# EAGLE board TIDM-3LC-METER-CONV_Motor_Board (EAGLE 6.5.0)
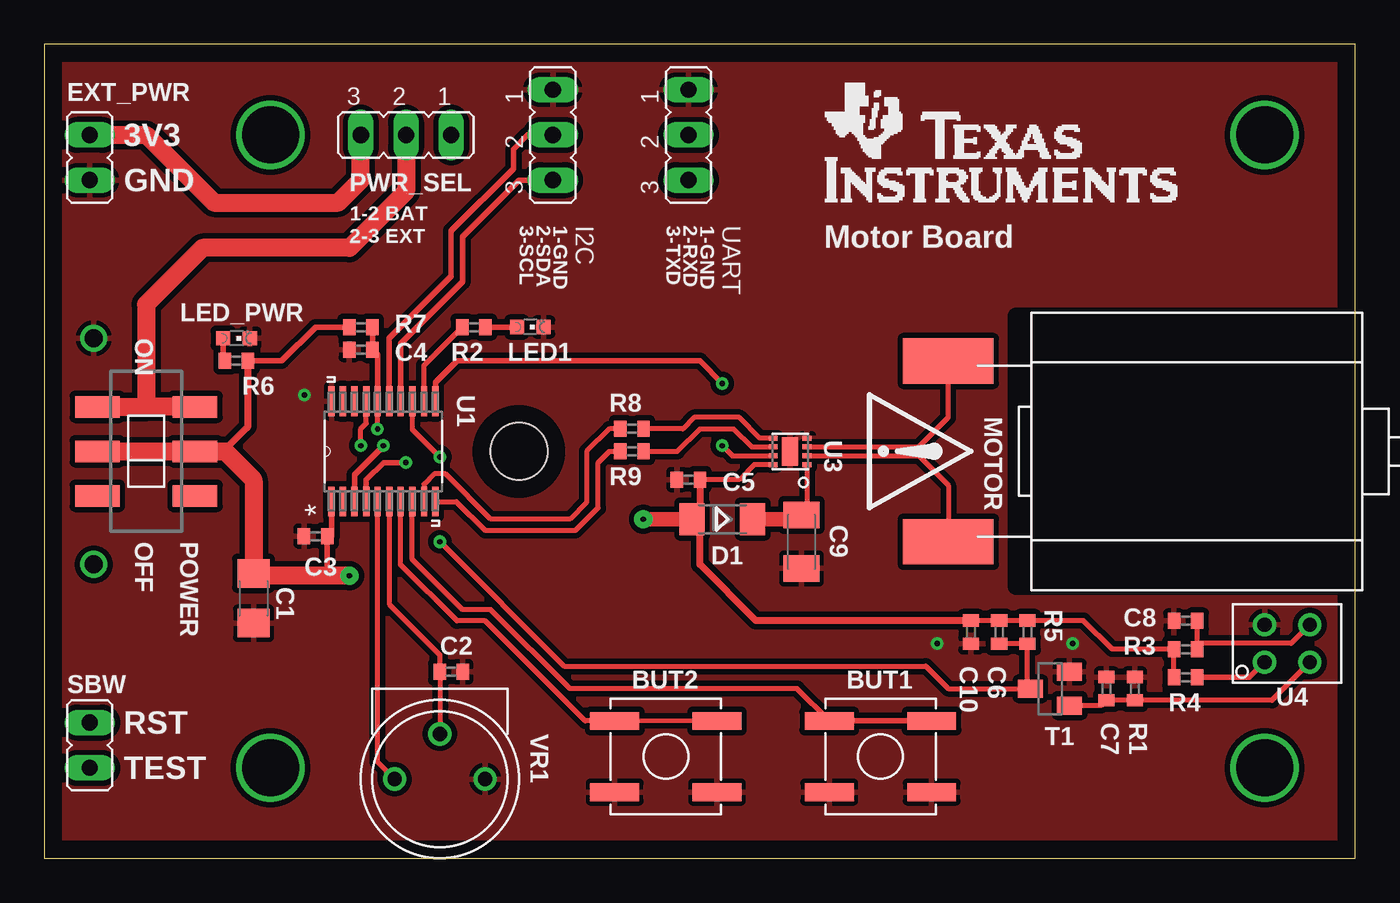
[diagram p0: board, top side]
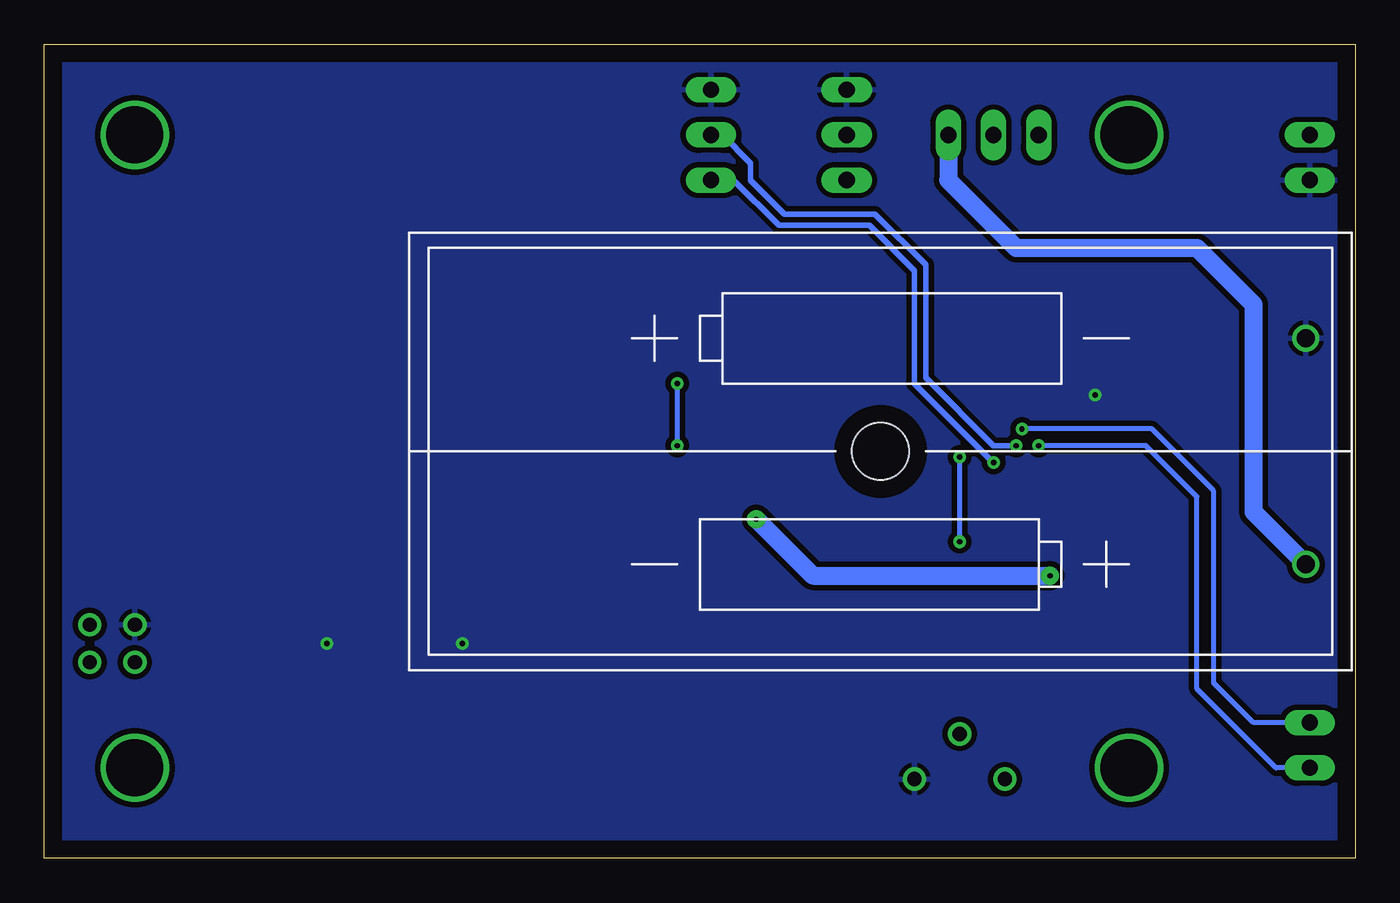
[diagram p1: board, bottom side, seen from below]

Size 73.66 x 45.72 mm. Coordinates in mm from the lower left corner, seen from the top.
Outline: 73.66,45.72 0,45.72 0,0 73.66,0 73.66,45.72
Copper layers (1*16): Top 0.035mm / dielectric 1.5mm / Bottom 0.035mm
Design rules "default *": minimum track width 6mil, minimum drill 0.3mm, track to track 6mil, track to pad 6mil, pad to pad 6mil, via to via 6mil, smd to smd 6mil, copper to edge 1mm, drill to drill 8mil, minimum pad ring 10mil, minimum via ring 8mil, stop-mask expansion 4mil, vias tented up to drill 100mil, thermal gap 10mil
tRestrict: area 54.6,15.2 to 73.7,30.5

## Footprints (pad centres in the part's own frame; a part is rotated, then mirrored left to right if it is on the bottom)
2X3A(1_HOLE) = drill 1: + 23.901,-6.35; - 23.901,6.35 | hole 3.2: 0,0
BUT = smd 2.75 x 1: P$1 2.875,-2; P$2 -2.875,-2; P$3 2.875,2; P$4 -2.875,2
C1206 = smd 1.6 x 1.8: 1 -1.4,0; 2 1.4,0
C0402 = smd 0.7 x 0.9: 1 -0.65,0; 2 0.65,0
C1206K = smd 1.5 x 2: 1 -1.5,0; 2 1.5,0
SOD80 = smd 1.4 x 1.8: 1 -1.7,0; 2 1.7,0
JP1 = drill 0.914 long: 1 0,-1.27; 2 0,1.27
JP2 = drill 0.914 long: 1 -2.54,0; 2 0,0; 3 2.54,0
CHIPLED_0603 = smd 0.8 x 0.8: A 0,-0.75; C 0,0.75
MOTOR = smd 5.08 x 2.54: + 13.97,5.08; - 13.97,-5.08
2P2T = smd 1.2 x 2.5: 1 -2.5,2.75; 2 0,2.75; 3 2.5,2.75; 4 -2.5,-2.75; 5 0,-2.75; 6 2.5,-2.75
R0402 = smd 0.7 x 0.9: 1 -0.65,0; 2 0.65,0
SOT23-BEC = smd 1 x 1.4: B -0.95,-1.1; C 0,1.1; E 0.95,-1.1
PW20 = smd 1.676 x 0.356: 1 -2.819,2.921; 2 -2.819,2.286; 3 -2.819,1.626; 4 -2.819,0.965; 5 -2.819,0.33; 6 -2.819,-0.33; 7 -2.819,-0.965; 8 -2.819,-1.626; 9 -2.819,-2.286; 10 -2.819,-2.921; 11 2.819,-2.921; 12 2.819,-2.286; 13 2.819,-1.626; 14 2.819,-0.965; 15 2.819,-0.33; 16 2.819,0.33; 17 2.819,0.965; 18 2.819,1.626; 19 2.819,2.286; 20 2.819,2.921
DSG-S-PWSON-N8 = smd 0.28 x 0.5: 1 -0.75,-0.95; 2 -0.25,-0.95; 3 0.25,-0.95; 4 0.75,-0.95; 5 0.75,0.95; 6 0.25,0.95; 7 -0.25,0.95; 8 -0.75,0.95 | smd 1.6 x 0.9: P$9 0,0
CUSTOM_4L = drill 0.8: P1 -1.054,1.27; P2 -1.054,-1.27; P3 1.054,-1.27; P4 1.054,1.27
3352P = drill 0.8: 1 -2.54,0; 2 0,-2.54; 3 2.54,0

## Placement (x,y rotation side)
BAT1  2XAAA-1  [2X3A(1_HOLE)]  26.67,22.86 0 bottom
BUT1  B3SL-1002P  [BUT]  46.99,5.71 0 top
BUT2  B3SL-1002P  [BUT]  34.92,5.71 0 top
C1  22uF  [C1206]  11.75,14.61 270 top
C2  100nF  [C0402]  22.86,10.48 0 top
C3  100nF  [C0402]  15.24,18.1 180 top
C4  2n2  [C0402]  17.78,28.57 180 top
C5  100nF  [C0402]  36.2,21.27 180 top
C6  470nF  [C0402]  53.66,12.7 270 top
C7  100nF  [C0402]  59.69,9.53 90 top
C8  100nF  [C0402]  64.14,13.34 180 top
C9  22uF  [C1206K]  42.55,17.78 270 top
C10  100nF  [C0402]  52.07,12.7 270 top
D1  FDLL4148  [SOD80]  38.1,19.05 180 top
EXT_PWR  [JP1]  2.54,39.37 180 top
I2C  [JP2]  28.57,40.64 270 top
LED1  [CHIPLED_0603]  27.3,29.84 270 top
LED_PWR  [CHIPLED_0603]  10.79,29.21 270 top
MOTOR  MOTOR  [MOTOR]  64.77,22.86 180 top
POWER  2P2T  [2P2T]  5.71,22.86 90 top
PWR_SEL  [JP2]  20.32,40.64 180 top
R1  10K  [R0402]  61.28,9.53 270 top
R2  470R  [R0402]  24.13,29.84 180 top
R3  1K  [R0402]  64.14,11.75 180 top
R4  100R  [R0402]  64.14,10.16 180 top
R5  2K  [R0402]  55.24,12.7 270 top
R6  470R  [R0402]  10.79,27.94 0 top
R7  47K  [R0402]  17.78,29.84 180 top
R8  100R  [R0402]  33.02,24.13 180 top
R9  100R  [R0402]  33.02,22.86 180 top
SBW  [JP1]  2.54,6.35 0 top
T1  [SOT23-BEC]  56.52,9.53 90 top
U1  MSP430G2333_PW_20  [PW20]  19.05,22.86 90 top
U3  DRV8837DSG  [DSG-S-PWSON-N8]  41.91,22.86 90 top
U4  QRD1113  [CUSTOM_4L]  69.85,12.06 90 top
U$1  TI-LOGO-SMALL  [TI-LOGO-4]  43.81,36.7 0 top
UART  [JP2]  36.2,40.64 270 top
VR1  3352P  [3352P]  22.23,4.45 180 top

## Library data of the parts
BAT1 = battery
BUT1 BUT2 = Button
C1-C10 R1-R9 = rcl
D1 = semicon-smd-ipc
EXT_PWR I2C PWR_SEL SBW UART = jumper
LED1 LED_PWR = led
MOTOR = motor
POWER = switch
T1 = transistor
U1 = MSP430; DATASHEETURL: http://www.ti.com/lit/gpn/MSP430G2333; DESCRIPTION: MSP430G2x33, MSP430G2x03 Mixed Signal Microcontroller; FAMILY_NAME: Value Line; GENERIC_PART_NUMBER: MSP430G2333; INDUSTRY_STD_PKG_TYPE: TSSOP; MANUFACTURER: Texas Instruments; MANUFACTURER_PART_NUMBER: msp430g2333_pw_20; PACKAGE_DESIGNATOR: PW; PIN_COUNT: 20; VENDOR: Texas Instruments
U3 = Motor Driver
U4 = Opto-Sensor
U$1 = texas-logo
VR1 = Trimmer

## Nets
BUT1: BUT1.P$3 BUT1.P$4 U1.8
BUT2: BUT2.P$3 BUT2.P$4 U1.7
GND: BAT1.- BUT1.P$1 BUT1.P$2 BUT2.P$1 BUT2.P$2 C1.2 C2.2 C3.2 C4.2 C5.2 C7.2 C8.2 C9.2 C10.2 EXT_PWR.2 I2C.1 LED1.C LED_PWR.C R1.1 T1.E U1.20 U3.4 U3.P$9 U4.P4 UART.1 VR1.1
LED: R2.2 U1.12
MOTOR_PWM1: R9.1 U3.6
MOTOR_PWM2: R8.1 U3.5
N$1: LED1.A R2.1
N$2: MOTOR.+ U3.2
N$3: C7.1 R1.2 T1.B U4.P2
N$4: MOTOR.- U3.3
N$5: R4.1 U4.P1
N$6: R8.2 U1.9
N$7: C9.1 D1.1 U3.1
N$8: R9.2 U1.10
N$10: C8.1 R3.1 U4.P3
N$13: BAT1.+ PWR_SEL.1
N$14: EXT_PWR.1 PWR_SEL.3
N$15: POWER.3 POWER.6 PWR_SEL.2
N$18: LED_PWR.A R6.1
ROT1: C6.2 R5.2 T1.C U1.13
RST/SBWTDIO: C4.1 R7.1 SBW.2 U1.16
RXD: U1.3 UART.2
SCL: I2C.3 U1.14
SDA: I2C.2 U1.15
SLEEP: U1.11 U3.7
TEST/SBWTCK: SBW.1 U1.17
TXD: U1.4 UART.3
VCC: C1.1 C3.1 C5.1 C6.1 C10.1 D1.2 POWER.2 POWER.5 R3.2 R4.2 R5.1 R6.2 R7.2 U1.1 U3.8
VRIN: C2.1 U1.6 VR1.2
VROUT: U1.5 VR1.3

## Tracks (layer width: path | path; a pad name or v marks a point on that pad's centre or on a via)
BUT1
  Top 0.279: BUT1.P$4 42.3,9.53 29.53,9.53 25.08,13.97 23.5,13.97 20.68,16.79 U1.8
  Top 0.305: BUT1.P$3 BUT1.P$4
BUT2
  Top 0.254: BUT2.P$4 BUT2.P$3 36.83,7.71
  Top 0.279: U1.7 20.02,16.5 23.18,13.34 24.77,13.34 30.39,7.71 BUT2.P$4
GND  (via drill 0.3)
  other vias: 50.16,12.06 57.78,12.06 14.61,26.04
  pour Bottom (isolate 0.305): 73.66,0 0,0 0,45.72 73.66,45.72
  pour Top (isolate 0.305): 73.66,45.72 0,45.72 0,0 73.66,0
LED
  Top 0.279: U1.12 21.34,27.69 R2.2
MOTOR_PWM1
  Top 0.279: R9.1 35.56,22.86 36.83,24.13 38.73,24.13 39.76,23.11 U3.6
MOTOR_PWM2
  Top 0.279: U3.5 40.21,23.61 39.05,24.77 36.51,24.77 35.88,24.13 R8.1
N$1
  Top 0.305: R2.1 LED1.A
N$2
  Top 0.279: U3.2 49.15,22.61 50.8,20.95 MOTOR.+
N$3
  Top 0.279: U4.P2 68.98,8.88 R1.2 C7.1 59.39,8.57 T1.B
N$4
  Top 0.279: U3.3 49.15,23.11 50.8,24.77 MOTOR.-
N$5
  Top 0.305: U4.P1 67.73,10.16 R4.1
N$6
  Top 0.279: R8.2 31.75,24.13 30.48,22.86 30.48,20 29.53,19.05 25.08,19.05 22.54,21.59 21.91,21.59 21.34,21.02 U1.9
N$7
  Top 0.279: U3.1 42.86,19.59 C9.1
  Top 0.813: D1.1 42.31,19.05 C9.1
N$8
  Top 0.279: U1.10 23.14,20.04 24.77,18.41 29.84,18.41 31.11,19.68 31.11,22.23 31.75,22.86 R9.2 32.38,22.84
N$10
  Top 0.279: C8.1 R3.1 64.78,12.06 70.07,12.06 U4.P3
N$13
  Bottom 1.016: PWR_SEL.1 22.86,38.1 19.05,34.29 8.89,34.29 5.71,31.11 5.71,19.46 BAT1.+
N$14
  Top 1.016: EXT_PWR.1 5.71,40.64 9.53,36.83 16.51,36.83 17.78,38.1 PWR_SEL.3
N$15
  Top 1.016: PWR_SEL.2 20.32,37.47 17.14,34.29 8.89,34.29 5.71,31.11 5.71,25.4 | 5.71,25.4 8.43,25.4 POWER.6 | POWER.3 5.67,25.36 5.71,25.4
N$16  (via drill 3.2)
  other vias: 12.7,40.64
N$17  (via drill 3.2)
  other vias: 12.7,5.08
N$18
  Top 0.305: R6.1 10.12,27.97 arc-45 10.04,28.14 LED_PWR.A
N$20  (via drill 3.2)
  other vias: 68.58,5.08
N$21  (via drill 3.2)
  other vias: 68.58,40.64
ROT1  (via drill 0.3)
  Top 0.279: C6.2 R5.2 55.24,9.7 T1.C 50.8,9.53 49.53,10.79 29.21,10.79 v22.23,17.78 | U1.13 20.68,24.09 v22.23,22.54
  Bottom 0.279: v22.23,22.54 v22.23,17.78
RST/SBWTDIO  (via drill 0.3)
  Top 0.279: v18.72,24.12 U1.16
  Top 0.305: U1.16 18.72,28.29 C4.1 R7.1
  Bottom 0.279: SBW.2 5.71,7.62 7.94,9.84 7.94,20.64 11.42,24.12 v18.72,24.12
RXD  (via drill 0.3)
  Top 0.305: v19.05,23.18 17.42,21.55 U1.3
  Bottom 0.305: v19.05,23.18 20.32,23.18 24.13,26.99 24.13,33.34 26.99,36.2 32.07,36.2 33.97,38.1 33.97,39.05 35.56,40.64 UART.2
SCL
  Top 0.305: U1.14 20.02,28.91 23.5,32.38 23.5,34.92 26.67,38.1 I2C.3
SDA
  Top 0.305: U1.15 19.38,29.22 22.86,32.7 22.86,35.24 26.35,38.73 26.35,39.85 27.15,40.64 I2C.2
SLEEP  (via drill 0.3)
  Top 0.279: v38.1,23.18 38.67,22.61 U3.7
  Top 0.305: U1.11 21.97,26.73 23.18,27.94 36.83,27.94 v38.1,26.67
  Bottom 0.279: v38.1,26.67 v38.1,23.18
TEST/SBWTCK  (via drill 0.3)
  Top 0.279: v17.78,23.18 17.78,24.13 18.09,24.43 U1.17
  Bottom 0.279: SBW.1 4.45,5.08 8.89,9.53 8.89,20.32 11.75,23.18 v17.78,23.18
TXD  (via drill 0.3)
  Top 0.305: v20.32,22.23 19.05,22.23 18.09,21.26 U1.4
  Bottom 0.305: UART.3 34.92,38.1 32.38,35.56 27.3,35.56 24.77,33.02 24.77,26.67 v20.32,22.23
VCC  (via drill 0.3 pad 1.02)
  Top 0.279: R4.2 R3.2 60.01,11.75 58.41,13.35 R5.1 C6.1 C10.1 | U3.8 39.89,22.11 39.05,21.27 C5.1
  Top 0.305: R6.2 13.34,27.94 15.24,29.84 R7.2 | U1.1 16.13,18.1 C3.1 15.88,18.1 15.88,15.88
  Top 0.406: C10.1 39.99,13.35 36.83,16.51 36.83,19.05 D1.2 36.84,19.05 C5.1 | 10.05,22.86 11.37,24.18 arc45 11.45,24.36 R6.2
  Top 0.813: v33.66,19.05 D1.2
  Top 1.016: POWER.2 POWER.5 10.05,22.86 arc-45 10.23,22.79 11.67,21.35 arc-45 11.75,21.17 C1.1 11.75,15.88 15.88,15.88 v17.14,15.88
  Bottom 1.016: v33.66,19.05 30.48,15.88 v17.14,15.88
VRIN
  Top 0.279: U1.6 19.38,14.28 22.21,11.45 C2.1 22.23,10.46 VR1.2
VROUT
  Top 0.279: VR1.3 18.72,5.41 U1.5

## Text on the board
tPlace: 3V3 | GND | 1-2 BAT | 3-SCL | 2-SDA | 1-GND | 3-TXD | 2-RXD | 1-GND | 2-3 EXT | Motor Board | ON | OFF | RST | TEST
